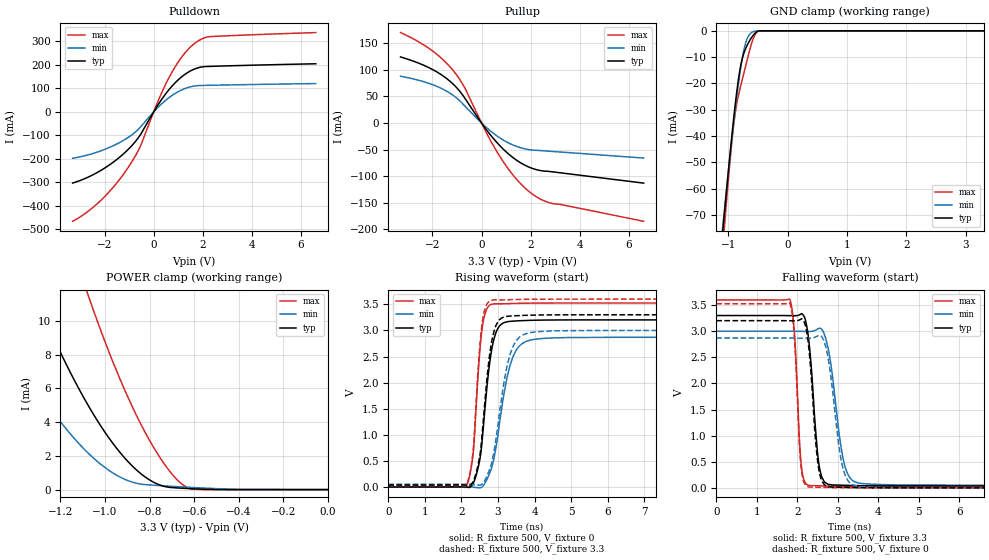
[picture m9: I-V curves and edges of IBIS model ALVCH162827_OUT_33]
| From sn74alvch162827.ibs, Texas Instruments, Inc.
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[Model]   ALVCH162827_OUT_33
Model_type  3-state
Enable   Active-Low
Vref =   0
Rref =   500
Cref =   50p
Vmeas =   1.5
| variable   typ   min   max
C_comp   7.11pF   6.22pF   8.40pF
| C_pullup   8.27pF   6.86pF   9.20pF
| C_pulldown   11.50pF   9.03pF   14.83pF
| C_tri-state   7.11pF   6.22pF   8.40pF
[Temperature Range]   40   100   -40
| Ambient temperature   25   85   -40
[Voltage range]   3.3   3   3.6
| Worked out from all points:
|   slope of the pulldown table from 0 to 0.495 V, typ, clamps not added: 6.36 ohm
|   slope of the pullup table from 0 to 0.495 V, typ, clamps not added: 16.5 ohm
|   GND clamp passes 1 mA (typ) near -0.55 V on its own axis
|   POWER clamp passes 1 mA (typ) near -0.84 V on its own axis
|   rising waveform, R_fixture 500, V_fixture 0: 20-80 % time 283ps typ, 421ps min, 201ps max; typ from 0 V to 3.2 V
|   falling waveform, R_fixture 500, V_fixture 3.3: 20-80 % time 190ps typ, 291ps min, 130ps max; typ from 3.3 V to 0.037 V
|   rising waveform, R_fixture 500, V_fixture 3.3: 20-80 % time 273ps typ, 399ps min, 198ps max; typ from 0.037 V to 3.3 V
|   falling waveform, R_fixture 500, V_fixture 0: 20-80 % time 184ps typ, 275ps min, 128ps max; typ from 3.2 V to 0 V
[GND Clamp]
| ALVCH162827_OUT_33
|   Voltage   I(typ)   I(min)   I(max)
-3.3V     -701.5mA   -639.5mA   -795.8mA
-1.09V    -75.9mA    -74.07mA   -82.03mA
-1.07V    -70.95mA   -69.58mA   -76.41mA
-1.05V    -66.05mA   -65.13mA   -70.87mA
-915mV    -34.94mA   -36.55mA   -37.33mA
-865mV    -24.93mA   -26.91mA   -28.93mA
-815mV    -16.6mA    -18.16mA   -23.39mA
-770mV    -11.23mA   -11.42mA   -19.2mA
-710mV    -6.971mA   -4.944mA   -13.82mA
-585mV    -1.88mA    -366.9uA   -3.413mA
-480mV    -19.21uA   -57.93uA   -14.88uA
3.3V      114.4pA    942nA      51.31pA
[POWER Clamp]
| ALVCH162827_OUT_33
|   Voltage   I(typ)   I(min)   I(max)
-3.3V     106mA      74.09mA    151.6mA
-1.545V   19.46mA    11.49mA    33.45mA
-1.32V    11.68mA    6.284mA    22.02mA
-1.295V   10.9mA     5.78mA     20.85mA
-1.195V   7.991mA    3.942mA    16.37mA
-1.075V   4.975mA    2.155mA    11.49mA
-965mV    2.743mA    987.8uA    7.581mA
-860mV    1.177mA    378.5uA    4.425mA
-760mV    302.3uA    241.6uA    2.031mA
-660mV    86.32uA    163.8uA    380.1uA
-605mV    48.5uA     124.6uA    22.06uA
-48.03fV  114.4pA    359.8pA    62.68pA
[Pulldown]
| ALVCH162827_OUT_33
|   Voltage   I(typ)   I(min)   I(max)
-3.3V     -302.4mA   -196.9mA   -465.1mA
-2.735V   -280.4mA   -184.4mA   -427.8mA
-2.16V    -249.3mA   -165.8mA   -377mA
-1.61V    -210.9mA   -141.8mA   -315.8mA
-1.105V   -166.3mA   -112.9mA   -246.6mA
-565mV    -100.8mA   -67.07mA   -151.3mA
185mV     31.43mA    20.51mA    47.78mA
665mV     100mA      64.12mA    153.8mA
1.17V     151.9mA    95.01mA    237.4mA
1.67V     182.8mA    110.5mA    291.9mA
2.31V     194mA      113.5mA    320.7mA
6.6V      205mA      120.8mA    337.8mA
[Pullup]
| ALVCH162827_OUT_33
|   Voltage   I(typ)   I(min)   I(max)
-3.3V     124.6mA    88.26mA    170.5mA
-2.055V   102.2mA    73.29mA    137.8mA
-1.565V   88.69mA    63.61mA    119.2mA
-1.15V    73.01mA    51.93mA    98.57mA
-690mV    47.45mA    32.47mA    66.81mA
180mV     -11.59mA   -7.766mA   -16.76mA
755mV     -43.3mA    -28.29mA   -63.76mA
1.375V    -68.47mA   -43.2mA    -103.3mA
1.995V    -84.31mA   -50.62mA   -131.4mA
2.4V      -89.62mA   -51.95mA   -143.5mA
2.81V     -91.58mA   -53.32mA   -150.8mA
6.6V      -113.3mA   -66.05mA   -185.3mA
[Ramp]
| ALVCH162827_OUT_33
| variable   typ   min   max
dV/dt_r   1.93/2.87E-10   1.73/4.32E-10   2.12/2.03E-10
dV/dt_f   1.98/1.98E-10   1.80/3.02E-10   2.15/1.35E-10
R_load = 500
[Rising Waveform]
| ALVCH162827_OUT_33
R_fixture =   500
C_fixture =   0
L_fixture =   0
V_fixture =   0
V_fixture_min = 0
V_fixture_max = 0
|   Time   V(typ)   V(min)   V(max)
0s        398pV      1.242nV    265.6pV
2.13ns    -2.979mV   3.841mV    9.93mV
2.325ns   70.96mV    -4.573mV   667.6mV
2.48ns    444.5mV    -16.79mV   2.392V
2.58ns    997.1mV    10.97mV    3.101V
2.745ns   2.221V     217.8mV    3.461V
2.895ns   2.847V     567.2mV    3.51V
3.415ns   3.178V     2.501V     3.517V
4.255ns   3.199V     2.848V     3.525V
50ns      3.202V     2.869V     3.526V
[Falling Waveform]
| ALVCH162827_OUT_33
R_fixture =   500
C_fixture =   0
L_fixture =   0
V_fixture =   3.3
V_fixture_min = 3
V_fixture_max = 3.6
|   Time   V(typ)   V(min)   V(max)
0s        3.3V       3V         3.6V
1.82ns    3.298V     3V         3.607V
1.93ns    3.296V     3V         2.988V
2.1ns     3.333V     2.998V     441.7mV
2.295ns   2.762V     2.994V     46.54mV
2.5ns     690.9mV    3.038V     40.81mV
2.61ns    204.6mV    3.032V     37.68mV
3.18ns    49.1mV     410.4mV    29.38mV
3.68ns    40.98mV    77.44mV    27.59mV
50ns      37.06mV    51.27mV    26.72mV
[Rising Waveform]
| ALVCH162827_OUT_33
R_fixture =   500
C_fixture =   0
L_fixture =   0
V_fixture =   3.3
V_fixture_min = 3
V_fixture_max = 3.6
|   Time   V(typ)   V(min)   V(max)
0s        37.06mV    51.27mV    26.72mV
2.13ns    33.35mV    54.38mV    37.1mV
2.325ns   111.5mV    45.28mV    725.4mV
2.47ns    475.6mV    34.97mV    2.398V
2.57ns    1.038V     58.2mV     3.155V
2.74ns    2.352V     279.9mV    3.539V
2.89ns    2.978V     672.4mV    3.586V
3.38ns    3.277V     2.638V     3.591V
4.16ns    3.296V     2.979V     3.599V
50ns      3.3V       3V         3.6V
[Falling Waveform]
| ALVCH162827_OUT_33
R_fixture =   500
C_fixture =   0
L_fixture =   0
V_fixture =   0
V_fixture_min = 0
V_fixture_max = 0
|   Time   V(typ)   V(min)   V(max)
0s        3.202V     2.869V     3.526V
1.82ns    3.2V       2.869V     3.532V
1.93ns    3.199V     2.868V     2.889V
2.095ns   3.232V     2.866V     402.1mV
2.29ns    2.658V     2.864V     16.03mV
2.475ns   728.2mV    2.897V     12.66mV
2.6ns     149.8mV    2.902V     9.731mV
3.14ns    10.47mV    351.6mV    2.524mV
3.585ns   3.846mV    22.32mV    918.9uV
50ns      242.4nV    -1.459nV   -1.229nV
